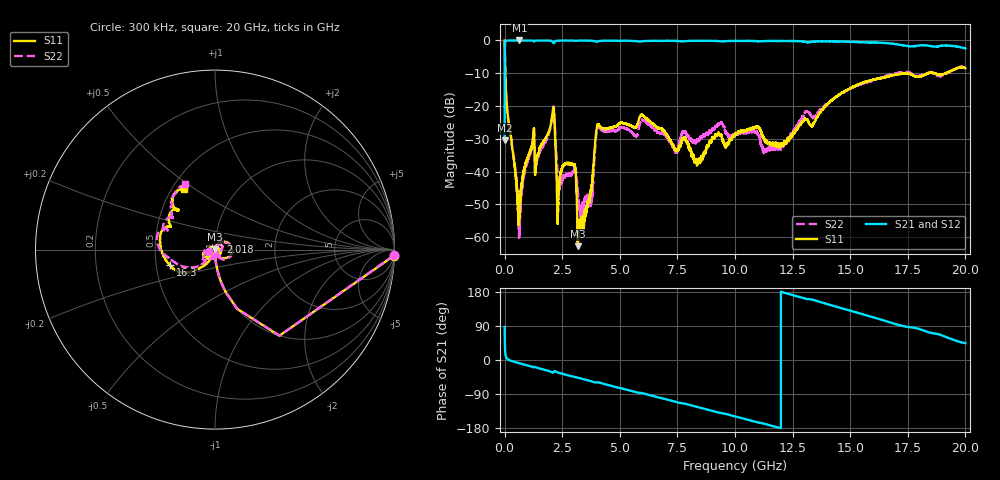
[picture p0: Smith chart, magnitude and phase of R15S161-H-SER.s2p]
!{R15S161}
!Johanson Technology Inc.
!www.johansontechnology.com
!Test Board Conditions:
!Substrate Type  RO4350B
!Substrate Thickness  20 mil
!Substrate Dk  3.66
!TL Type: GCPW
!TL Trace Width  34 mil
!TL Gap  10 mil
!Electrode orientation  Horizontal
!DUT TOPOLOGY	SERIES
!Mounting Pad LxW  26x52 mil
! Created Sat Feb  6 14:16:09 2021
# hz S ma R 50
! 2 Port Network Data from SP1.SP block
! freq  magS11  angS11  magS21  angS21  magS12  angS12  magS22  angS22
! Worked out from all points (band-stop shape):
!   20001 points, 300 kHz to 20 GHz, reference 50 ohm
!   highest |S21| = -0.01 dB at 643.3 MHz (marker M1); lowest = -30.4 dB at 300 kHz (marker M2)
!   |S21| within 3 dB of the highest: 10.03 MHz to end of sweep
!   lowest |S11| = -62.7 dB at 3.183 GHz (marker M3), VSWR 1.00, Z = 50 + j0.0574 ohm
!   |S11| at or under -10 dB: 29.77 MHz to 17.34 GHz (17.31 GHz wide, 199 % of centre); 17.48 GHz to 18.39 GHz (908.4 MHz wide, 5.06 % of centre); 18.71 GHz to 19.15 GHz (440.5 MHz wide, 2.33 % of centre)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
!   |S22| runs from -60.2 to 0.0 dB; largest |S21 - S12| = 0.017
!   S11 on the Smith chart (normalised r, x): 300 kHz: 5, -57; 2.018 GHz: 1.07, +0.09; 16.3 GHz: 0.59, -0.11; 20 GHz: 0.58, +0.45
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300000  0.9968 -2.0  0.03012 87.5  0.03015 87.9  0.9972 -1.8
1.073e8  0.09107 -85.0  0.993 3.7  0.9938 3.7  0.09173 -84.9
6.433e8  0.002432 28.8  0.9986 -8.8  0.9972 -8.7  0.00137 5.9
1.1923e9  0.02586 67.9  0.9951 -17.8  0.9956 -17.8  0.02433 67.3
1.4043e9  0.01616 67.2  0.9955 -20.4  0.9956 -20.3  0.01466 60.9
2.0183e9  0.05491 51.4  0.9856 -31.4  0.9844 -31.4  0.05181 44.6
2.1383e9  0.08663 -26.7  0.9059 -30.5  0.9059 -30.5  0.09259 -28.7
2.3293e9  0.003316 52.2  0.9908 -33.2  0.9914 -33.2  0.006863 -41.2
2.9743e9  0.01284 52.6  0.9927 -44.0  0.993 -44.0  0.009713 28.8
3.1833e9  0.0007323 51.6  0.9913 -46.7  0.9922 -46.7  0.004768 -70.3
3.3343e9  0.001802 125.7  0.9938 -49.2  0.9934 -49.1  0.002087 -123.0
3.7533e9  0.005334 -89.4  0.9898 -56.1  0.9892 -56.1  0.003598 -107.3
4.0693e9  0.05241 -118.6  0.9669 -58.9  0.9664 -59.0  0.04857 -120.5
6.6673e9  0.04628 -170.4  0.9847 -98.6  0.985 -98.6  0.03913 175.9
7.4383e9  0.02158 -155.3  0.9811 -110.5  0.9828 -110.6  0.01997 -175.4
8.3983e9  0.01466 63.2  0.9869 -124.6  0.9852 -124.5  0.02954 -124.7
1.00003e10  0.037 -63.1  0.9835 -148.8  0.9828 -148.8  0.03653 -72.9
1.19223e10  0.02477 -117.0  0.9794 -178.9  0.9796 -178.9  0.024 -75.8
1.33343e10  0.04949 -126.5  0.95 159.7  0.9501 159.6  0.06733 -143.2
1.63043e10  0.2644 -160.7  0.9225 107.2  0.916 107.3  0.2687 -170.5
1.66673e10  0.2811 -170.3  0.9073 100.3  0.8927 100.3  0.2968 -176.9
2e10  0.3777 117.2  0.7595 44.8  0.7522 44.7  0.3994 114.2
